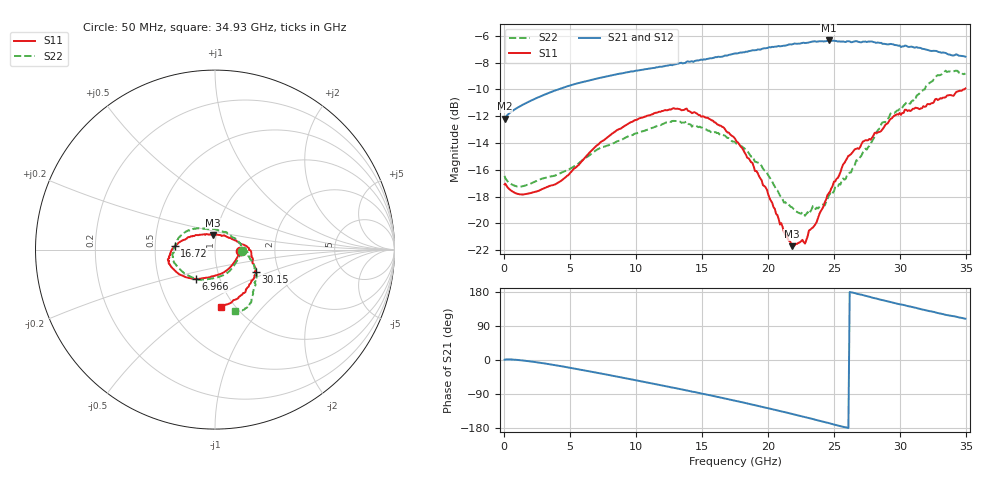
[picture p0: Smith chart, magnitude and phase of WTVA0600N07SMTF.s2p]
! 50 ohm 2-Port S-parameters measured by Modelithics Inc support@modelithics.com  Tampa, FL USA 813-866-6335 (February 2024)
! Smiths Interconnect,  6dB P/N: WTVA0600N07SMTF, Temperature: -50 C
! Board: 10 mil Rogers 4350B, Mounting Pad Dimensions: Length: 15 mils, Width: 25 mils, Gap: 40 mils.
# Hz S RI R 50
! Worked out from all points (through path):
!   352 points, 50 MHz to 34.93 GHz, reference 50 ohm
!   highest |S21| = -6.35 dB at 24.58 GHz (marker M1); lowest = -12.2 dB at 50 MHz (marker M2)
!   group delay of S21, straight-line fit = 21.1 ps
!   lowest |S11| = -21.7 dB at 21.79 GHz (marker M3), VSWR 1.18, Z = 48.3 + j7.95 ohm
!   |S11| at or under -10 dB: start of sweep to 34.83 GHz
!   |S22| runs from -19.4 to -8.6 dB; largest |S21 - S12| = 0.0029
!   S11 on the Smith chart (normalised r, x): 50 MHz: 1.32, -0.02; 6.966 GHz: 0.77, -0.26; 16.72 GHz: 0.63, +0.03; 30.15 GHz: 1.52, -0.40; 34.93 GHz: 0.87, -0.61
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5e7  0.1398 -0.00576  0.2461 0.00353  0.2459 0.00345  0.1503 -0.00587
9.96e8  0.1143 -0.0601  0.2697 0.00137  0.2694 0.00139  0.1216 -0.064
2.4885e9  0.0705 -0.1112  0.2922 -0.0309  0.2919 -0.0309  0.0806 -0.1195
4.18e9  0.00947 -0.1423  0.3056 -0.0845  0.3054 -0.0844  0.0236 -0.1515
5.8715e9  -0.0611 -0.1588  0.3019 -0.1478  0.3016 -0.1477  -0.0432 -0.1658
6.966e9  -0.1045 -0.1636  0.2898 -0.1896  0.2896 -0.1893  -0.0828 -0.1682
1.1742e10  -0.2421 -0.098  0.1582 -0.3498  0.1576 -0.3497  -0.2157 -0.0874
1.38315e10  -0.2629 -0.0538  0.0693 -0.3953  0.0692 -0.3951  -0.2384 -0.0285
1.6717e10  -0.2242 0.0203  -0.0833 -0.4147  -0.0837 -0.4144  -0.202 0.0667
1.7513e10  -0.2026 0.039  -0.1301 -0.4109  -0.1303 -0.4106  -0.1809 0.0874
1.9901e10  -0.1063 0.0812  -0.2685 -0.3625  -0.2682 -0.3624  -0.0981 0.1192
2.11945e10  -0.0392 0.084  -0.3376 -0.3129  -0.3378 -0.3124  -0.0376 0.1135
2.17915e10  -0.0103 0.0816  -0.3676 -0.2853  -0.3675 -0.2851  -0.00986 0.1147
2.27865e10  0.0366 0.0757  -0.4112 -0.2294  -0.4112 -0.2289  0.0358 0.1008
2.33835e10  0.0634 0.0728  -0.4349 -0.1959  -0.4349 -0.1954  0.0608 0.0989
2.4279e10  0.1067 0.0544  -0.459 -0.1327  -0.459 -0.1322  0.0939 0.0692
2.45775e10  0.1205 0.0473  -0.468 -0.113  -0.4679 -0.1125  0.1093 0.0636
2.607e10  0.1777 0.0177  -0.4779 -0.00381  -0.4776 -0.00342  0.1518 0.0223
2.91545e10  0.2218 -0.0949  -0.419 0.2041  -0.4185 0.2046  0.2254 -0.1077
3.01495e10  0.2273 -0.1227  -0.3796 0.2555  -0.3792 0.2556  0.2315 -0.1397
3.3433e10  0.1318 -0.2648  -0.2103 0.3777  -0.2101 0.3775  0.1888 -0.3197
3.49255e10  0.033 -0.317  -0.1361 0.3961  -0.1342 0.3965  0.113 -0.3447
